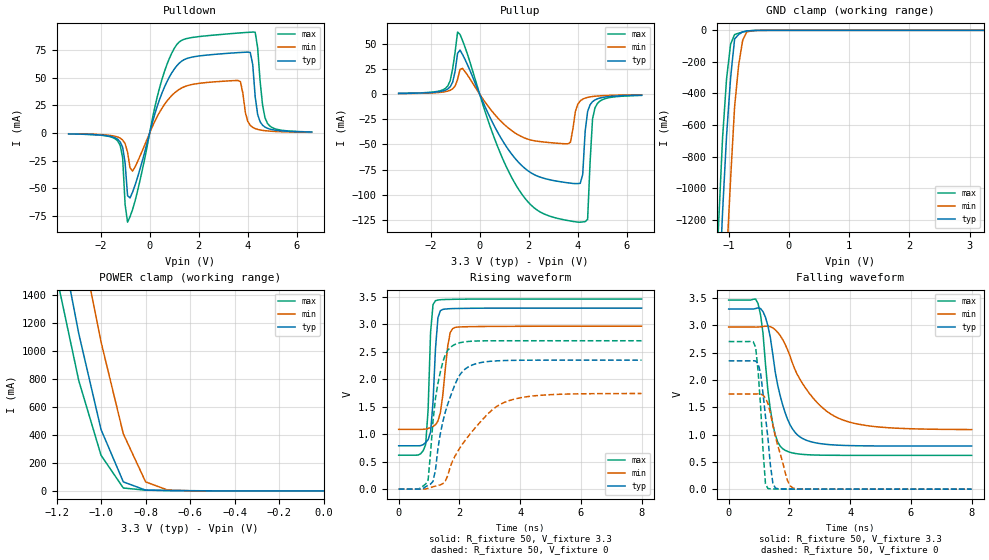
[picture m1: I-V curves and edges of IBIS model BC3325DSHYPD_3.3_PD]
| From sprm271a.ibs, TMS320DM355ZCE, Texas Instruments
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|   Component BC3325DSHYPD
|   Model Cell BC3325DSHYPD_3.3_PD
[Model]   BC3325DSHYPD_3.3_PD
Model_type   I/O
Polarity   Non-Inverting
Enable   Active-Low
Vinl =  1.5
Vinh =  1.8
Cref =  15.0000pF
Rref =  100.0000M
Vref =  0V
Vmeas =  1.65
C_comp   0.972592p   0.9599789p   0.9808023p
[Model Spec]
Vinl   1.5   1.335   1.5825
Vinh   1.8   1.635   1.8825
[Temperature Range]   25   125   -40
[Voltage Range]   3.3   2.97   3.465
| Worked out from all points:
|   slope of the pulldown table from 0 to 0.495 V, typ, clamps not added: 13.9 ohm
|   slope of the pullup table from 0 to 0.495 V, typ, clamps not added: 18.5 ohm
|   GND clamp passes 1 mA (typ) near -0.58 V on its own axis
|   POWER clamp passes 1 mA (typ) near -0.54 V on its own axis
|   rising waveform, R_fixture 50, V_fixture 3.3: 20-80 % time 159ps typ, 222ps min, 120ps max; typ from 0.79 V to 3.3 V
|   rising waveform, R_fixture 50, V_fixture 0: 20-80 % time 599ps typ, 1.31ns min, 355ps max; typ from 0 V to 2.35 V
|   falling waveform, R_fixture 50, V_fixture 3.3: 20-80 % time 566ps typ, 1.23ns min, 333ps max; typ from 3.3 V to 0.79 V
|   falling waveform, R_fixture 50, V_fixture 0: 20-80 % time 266ps typ, 468ps min, 186ps max; typ from 2.35 V to 0 V
[POWER_clamp]
|   voltage   I(typ)   I(min)   I(max)
-3.3V     22.26A     22.98A     21.87A
-1.2V     1.951A     2.729A     1.539A
-1.167V   1.675A     2.441A     1.289A
-1.133V   1.4A       2.153A     1.039A
-1.1V     1.125A     1.865A     788.5mA
-1.067V   896.1mA    1.599A     610.6mA
-1.033V   667.5mA    1.332A     432.7mA
-1V       438.9mA    1.066A     254.8mA
-900mV    64.53mA    408.4mA    20.87mA
-800mV    5.881mA    64.81mA    5.363mA
-700mV    2.694mA    5.859mA    3.293mA
-11.55fV  98.21uA    49.4uA     162.3uA
[Pulldown]
|   voltage   I(typ)   I(min)   I(max)
-3.3V     -808.1uA   -658.5uA   -838.6uA
-1.3V     -5.711mA   -3.626mA   -7.219mA
-1.1V     -12.9mA    -6.318mA   -22.43mA
-900mV    -56.47mA   -17.38mA   -80.42mA
-700mV    -53.51mA   -34.37mA   -69.3mA
400mV     30mA       18.55mA    40.42mA
1.1V      60.43mA    37.7mA     79.59mA
3.7V      72.61mA    46.35mA    90.3mA
4.2V      61.81mA    5.119mA    91.01mA
4.4V      16.79mA    3.291mA    77.11mA
4.8V      4.264mA    1.885mA    8.735mA
6.6V      871.4uA    628.5uA    963.3uA
[Pullup]
|   voltage   I(typ)   I(min)   I(max)
-3.3V     659.6uA    522.1uA    739.6uA
-1.3V     5.125mA    2.966mA    8.081mA
-900mV    40.49mA    14.5mA     61.66mA
-700mV    39.49mA    25.52mA    53.37mA
1.6V      -68.17mA   -40.92mA   -95.13mA
3.6V      -88.21mA   -49.34mA   -125.7mA
4.1V      -88.68mA   -6.718mA   -127.3mA
4.2V      -79.9mA    -4.993mA   -127mA
4.4V      -17.25mA   -3.255mA   -124.4mA
4.6V      -7.503mA   -2.398mA   -24.77mA
4.7V      -5.775mA   -2.116mA   -13.67mA
6.6V      -1.03mA    -644.3uA   -1.277mA
[GND_clamp]
|   voltage   I(typ)   I(min)   I(max)
-3.3V     -22.38A    -23.15A    -21.96A
-1.167V   -1.724A    -2.574A    -1.236A
-1.1V     -1.154A    -1.991A    -682.8mA
-1.033V   -667.2mA   -1.446A    -306.3mA
-966.7mV  -300.6mA   -943.8mA   -87.48mA
-900mV    -54.67mA   -483.6mA   -26.51mA
-833.3mV  -26.38mA   -221.3mA   -17.72mA
-766.7mV  -9.699mA   -63.68mA   -10.38mA
-700mV    -4.619mA   -10.64mA   -4.488mA
-566.7mV  -733.7uA   -1.505mA   -501.4uA
-433.3mV  -74.6uA    -170uA     -70.9uA
3.233V    98.2uA     61.66uA    162.2uA
[Ramp]
| variable   typ   min   max
dV/dt_f   1.518725/0.5668402n   1.136924/1.233969n   1.721499/0.3331091n
dV/dt_r   1.410457/0.6004938n   1.04586/1.315014n   1.622549/0.3476211n
R_load = 50
[Rising Waveform]
R_fixture = 50
V_fixture = 3.3
V_fixture_min = 2.97
V_fixture_max = 3.465
| time   V(typ)   V(min)   V(max)
|   time   V(typ)   V(min)   V(max)
0s        790mV      1.089V     619mV
888.9ps   849.4mV    1.094V     811mV
969.7ps   900.9mV    1.105V     1.451V
1.051ns   1.038V     1.123V     2.857V
1.212ns   2.555V     1.172V     3.434V
1.293ns   3.124V     1.24V      3.446V
1.374ns   3.252V     1.394V     3.451V
1.616ns   3.286V     2.608V     3.457V
1.859ns   3.291V     2.947V     3.46V
8ns       3.299V     2.969V     3.463V
[Rising Waveform]
R_fixture = 50
V_fixture = 0
V_fixture_min = 0
V_fixture_max = 0
| time   V(typ)   V(min)   V(max)
|   time   V(typ)   V(min)   V(max)
0s        34.13nV    295.4nV    3.062nV
646.5ps   -562uV     -213.3uV   2.583mV
969.7ps   70.31mV    13.08mV    168.3mV
1.131ns   142.4mV    43.23mV    1.249V
1.293ns   740.6mV    65.56mV    1.926V
1.535ns   1.404V     149.4mV    2.451V
1.778ns   1.799V     516.6mV    2.614V
2.343ns   2.242V     999.5mV    2.693V
3.556ns   2.344V     1.597V     2.704V
8ns       2.35V      1.742V     2.704V
[Falling Waveform]
R_fixture = 50
V_fixture = 3.3
V_fixture_min = 2.97
V_fixture_max = 3.465
| time   V(typ)   V(min)   V(max)
|   time   V(typ)   V(min)   V(max)
0s        3.299V     2.969V     3.463V
969.7ps   3.32V      2.969V     3.395V
1.131ns   3.25V      2.979V     2.852V
1.212ns   3.147V     2.985V     2.288V
1.455ns   2.463V     2.953V     1.186V
1.616ns   1.901V     2.871V     863.4mV
1.859ns   1.4V       2.653V     712.3mV
2.586ns   890.2mV    1.809V     631.1mV
3.636ns   804.9mV    1.295V     619.8mV
8ns       790mV      1.092V     619mV
[Falling Waveform]
R_fixture = 50
V_fixture = 0
V_fixture_min = 0
V_fixture_max = 0
| time   V(typ)   V(min)   V(max)
|   time   V(typ)   V(min)   V(max)
0s        2.35V      1.743V     2.704V
888.9ps   2.348V     1.743V     2.597V
969.7ps   2.295V     1.746V     2.157V
1.051ns   2.127V     1.744V     1.525V
1.212ns   1.332V     1.667V     96.91mV
1.293ns   935.8mV    1.566V     11.7mV
1.455ns   111.9mV    1.176V     3.696mV
1.939ns   2.625mV    153.6mV    1.051mV
2.101ns   1.943mV    24.94mV    717.9uV
8ns       389.5nV    12.56uV    152.9nV
